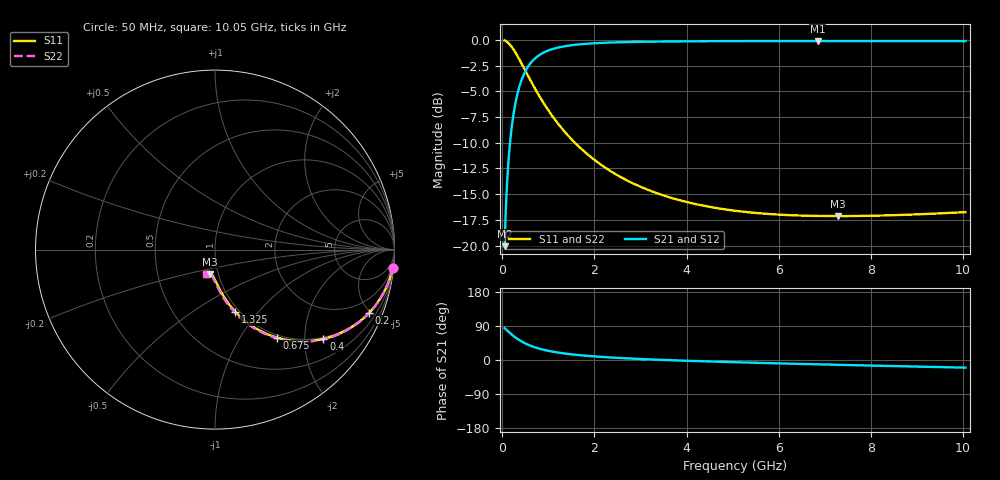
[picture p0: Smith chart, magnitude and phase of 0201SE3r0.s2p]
! AVX Thin Film Operation		Date: August 2001
! Description: Accu-P® Series, Thin Film, SMD, RF Capacitor
! Part Number: 0201YJ3R0ABW
! 50 MHz  -  10.05 GHz
! Serial Measurements
# mhz S db R 50
!	S11		S21		S12		S22
!	dB	Phase	dB	Phase	dB	Phase	dB	Phase
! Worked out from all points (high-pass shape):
!   401 points, 50 MHz to 10.05 GHz, reference 50 ohm
!   highest |S21| = -0.09 dB at 6.85 GHz (marker M1); lowest = -20.1 dB at 50 MHz (marker M2)
!   |S21| within 3 dB of the highest: 494.7 MHz to end of sweep
!   lowest |S11| = -17.1 dB at 7.275 GHz (marker M3), VSWR 1.32, Z = 45.7 - j12.7 ohm
!   |S11| at or under -10 dB: 1.577 GHz to end of sweep
!   |S22| runs from -17.1 to 0.0 dB; largest |S21 - S12| = 0
!   S11 on the Smith chart (normalised r, x): 50 MHz: 1, -20; 200 MHz: 0.96, -4.91; 400 MHz: 0.96, -2.46; 675 MHz: 0.96, -1.46; 1.325 GHz: 0.96, -0.76; 10.05 GHz: 0.88, -0.25
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50  -0.04 -5.8  -20.06 84.2  -20.06 84.2  -0.04 -5.9
75  -0.10 -8.7  -16.59 81.3  -16.59 81.3  -0.10 -8.8
125  -0.26 -14.3  -12.33 75.6  -12.33 75.6  -0.26 -14.4
150  -0.37 -17.0  -10.86 72.9  -10.86 72.9  -0.37 -17.1
200  -0.64 -22.2  -8.63 67.7  -8.63 67.7  -0.64 -22.4
250  -0.97 -27.1  -7.02 62.8  -7.02 62.8  -0.96 -27.3
300  -1.33 -31.6  -5.80 58.3  -5.80 58.3  -1.33 -31.8
400  -2.13 -39.5  -4.12 50.3  -4.12 50.3  -2.13 -39.8
525  -3.20 -47.5  -2.84 42.3  -2.84 42.3  -3.20 -47.8
675  -4.45 -54.9  -1.94 34.9  -1.94 34.9  -4.45 -55.3
800  -5.43 -59.6  -1.48 30.1  -1.48 30.1  -5.43 -60.1
950  -6.51 -64.1  -1.11 25.5  -1.11 25.5  -6.51 -64.7
1325  -8.77 -71.9  -0.63 17.6  -0.63 17.6  -8.77 -72.7
1725  -10.63 -77.2  -0.40 12.2  -0.40 12.2  -10.63 -78.2
2500  -13.16 -83.6  -0.22 5.6  -0.22 5.6  -13.16 -85.0
3400  -14.98 -88.3  -0.15 0.6  -0.15 0.6  -14.98 -90.1
5050  -16.61 -94.5  -0.10 -5.9  -0.10 -5.9  -16.62 -96.6
6725  -17.11 -99.6  -0.09 -11.1  -0.09 -11.1  -17.11 -101.7
6850  -17.12 -99.9  -0.09 -11.5  -0.09 -11.5  -17.12 -102.1
7275  -17.14 -101.1  -0.09 -12.7  -0.09 -12.7  -17.14 -103.3
8400  -17.06 -104.2  -0.10 -15.8  -0.10 -15.8  -17.06 -106.3
10050  -16.75 -108.6  -0.10 -20.2  -0.10 -20.2  -16.75 -110.6
